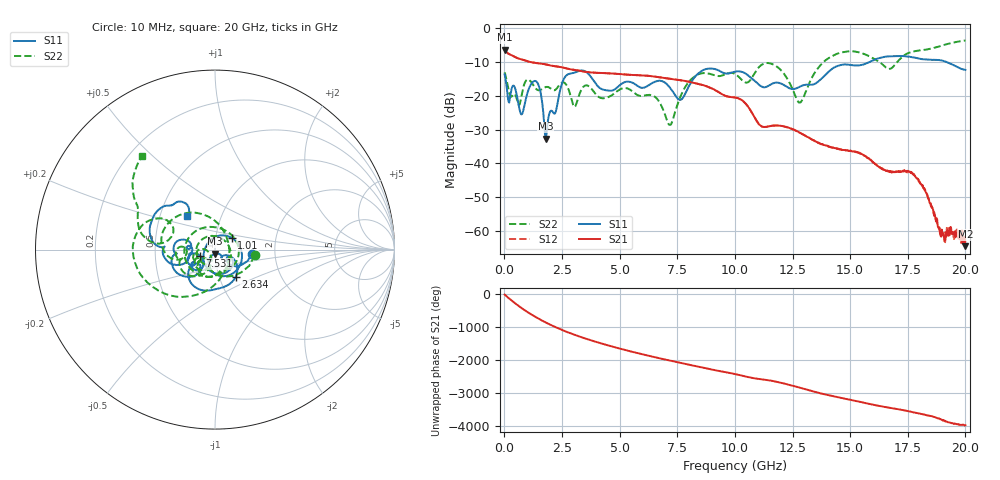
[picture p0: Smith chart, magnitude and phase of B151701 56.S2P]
!  2-Port S-parameters saved by WinCal
! VAR MeasName=S-Parameters (CALIBRATED_DATA) read from VNA (N5244A)
! VAR MeasDate=2015-12-24 19:16:28
! VAR NAME=B151701 56
! VAR FILENAME=B151701 56.S2P
! VAR DATE=2015-12-24 19:16:28
! VAR PHYS_PORTS=1,3
# Hz S DB R 50
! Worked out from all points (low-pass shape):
!   801 points, 10 MHz to 20 GHz, reference 50 ohm
!   highest |S21| = -6.28 dB at 10 MHz (marker M1); lowest = -64.5 dB at 20 GHz (marker M2)
!   |S21| within 3 dB of the highest: start of sweep to 796.2 MHz
!   lowest |S11| = -32.7 dB at 1.784 GHz (marker M3), VSWR 1.05, Z = 50 - j2.33 ohm
!   |S11| at or under -10 dB: start of sweep to 15.83 GHz; 19.2 GHz to end of sweep
!   |S22| runs from -28.6 to -3.6 dB; largest |S21 - S12| = 0.0011
!   S11 on the Smith chart (normalised r, x): 10 MHz: 1.52, -0.07; 1.01 GHz: 1.19, +0.16; 2.634 GHz: 1.19, -0.38; 7.531 GHz: 0.84, -0.06; 20 GHz: 0.69, +0.27
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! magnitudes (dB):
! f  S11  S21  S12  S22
! 10 MHz  -13.6  -6.3  -6.3  -13.0
! 609.7 MHz  -22.4  -8.9  -8.9  -22.6
! 1.01 GHz  -18.9  -9.8  -9.7  -15.2
! 1.434 GHz  -16.1  -10.3  -10.3  -18.2
! 1.784 GHz  -32.7  -10.7  -10.7  -17.4
! 2.634 GHz  -14.4  -11.8  -11.8  -16.3
! 3.033 GHz  -13.1  -12.3  -12.3  -23.2
! 3.358 GHz  -12.5  -12.7  -12.7  -17.9
! 4.508 GHz  -18.4  -13.3  -13.3  -20.4
! 6.682 GHz  -15.6  -14.4  -14.4  -21.4
! 7.181 GHz  -17.6  -14.9  -14.9  -28.6
! 7.531 GHz  -20.8  -15.2  -15.2  -22.1
! 8.381 GHz  -13.5  -16.4  -16.4  -13.7
! 10.01 GHz  -12.8  -20.5  -20.5  -13.5
! 11.63 GHz  -16.4  -28.8  -28.8  -10.6
! 12.8 GHz  -17.3  -30.9  -30.9  -22.0
! 13.35 GHz  -16.7  -33.0  -33.0  -14.4
! 14.88 GHz  -10.7  -36.1  -36.1  -6.8
! 16.68 GHz  -8.3  -42.4  -42.3  -12.0
! 17.75 GHz  -8.6  -43.4  -43.3  -6.8
! 19.03 GHz  -9.6  -60.8  -61.2  -5.0
! 20 GHz  -12.3  -64.5  -63.4  -3.6
